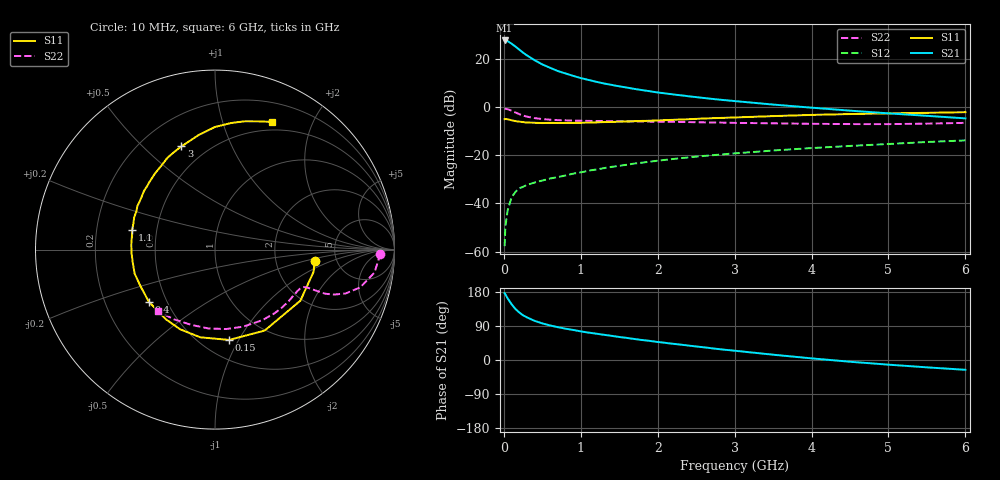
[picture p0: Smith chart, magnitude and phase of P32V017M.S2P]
! SIEMENS Small Signal Semiconductors
! BFP181
! Si NPN RF Bipolar Junction Transistor in SOT143
! VCE = 2 V  IC = 17 mA
! Common Emitter S-Parameters:  March  1996
# GHz  S  MA  R  50
!  f  S11  S21  S12  S22
! GHz  MAG  ANG  MAG  ANG  MAG  ANG  MAG  ANG
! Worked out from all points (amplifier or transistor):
!   36 points, 10 MHz to 6 GHz, reference 50 ohm
!   highest |S21| = 27.6 dB at 10 MHz (marker M1)
!   |S21| within 3 dB of that: start of sweep to 169.3 MHz
!   unconditionally stable (mu >= 1): start of sweep to 15.18 MHz; 437.4 MHz to end of sweep
!   at 250 MHz: K = 0.69, MSG = 27.8 dB, |S12| = -33.1 dB
!   at 1.4 GHz: K = 1.57, MAG = 12.5 dB, |S12| = -24.9 dB
!   at 6 GHz: K = 1.22, MAG = 1.8 dB, |S12| = -13.9 dB
!   S11 on the Smith chart (normalised r, x): 10 MHz: 3.41, -0.62; 150 MHz: 0.67, -0.91; 400 MHz: 0.40, -0.30; 1.1 GHz: 0.36, +0.10; 3 GHz: 0.36, +0.66; 6 GHz: 0.40, +1.46
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0.01  0.5585 -6.4  23.85 176.4  0.0013 79.5  0.9222 -1.4
0.02  0.563 -12.7  23.8 173.2  0.0033 84.3  0.914 -3.2
0.05  0.5543 -30.9  23.06 162.4  0.0072 81.2  0.8978 -8.2
0.1  0.5293 -58.5  20.48 147.2  0.0133 64.5  0.8359 -14.6
0.15  0.5094 -81.1  17.86 134.8  0.0173 58.1  0.7669 -18.6
0.2  0.4955 -99.5  15.45 125.4  0.0206 53.9  0.7091 -20.7
0.25  0.4847 -113.6  13.32 117.9  0.0221 51.5  0.6625 -21.8
0.3  0.475 -125.0  11.71 112.5  0.0242 50.2  0.6297 -22.0
0.4  0.4695 -141.7  9.298 103.3  0.0271 49.3  0.5859 -22.2
0.5  0.4625 -154.0  7.594 96.6  0.0298 49.3  0.5597 -22.3
0.6  0.4672 -163.3  6.475 91.2  0.0328 50.6  0.5435 -22.6
0.7  0.4639 -171.1  5.558 86.7  0.0351 51.3  0.5333 -23.1
0.9  0.4674 176.6  4.413 79.3  0.0414 53.6  0.521 -24.7
1.1  0.474 166.5  3.628 72.3  0.0476 54.8  0.5132 -26.9
1.5  0.4958 150.8  2.672 60.7  0.06 55.1  0.5041 -32.3
1.8  0.5134 140.4  2.228 52.7  0.07 54.6  0.4981 -37.1
2.2  0.5403 128.2  1.818 42.8  0.0835 52.7  0.4891 -43.9
3  0.6047 108.0  1.323 24.5  0.1089 47.7  0.4676 -59.2
3.5  0.6449 98.1  1.119 14.0  0.1249 44.3  0.457 -70.1
4.5  0.7116 82.6  0.837 -4.6  0.1553 36.2  0.4408 -94.9
5.5  0.7543 71.3  0.654 -19.4  0.1875 28.3  0.4504 -120.2
6  0.7781 66.1  0.579 -25.9  0.2023 23.5  0.4676 -132.5
